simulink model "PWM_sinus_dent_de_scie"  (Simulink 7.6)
settings: Solver=ode15s  StartTime=0.0  StopTime=0.02  RelTol=1e-3
StopFcn:
  | close all, clc
  | load signaux.mat
  | plot(x(1,:),x(2,:),x(1,:),x(3,:),x(1,:),x(4,:))
  | title('Signal PWM, sinus et dent de scie')
  | axis([0 0.02 -2 6])
  | xlabel('temps')
  | grid
libraries: fl_lib x10, nesl_utility x6, elec_lib x1, simulink x1

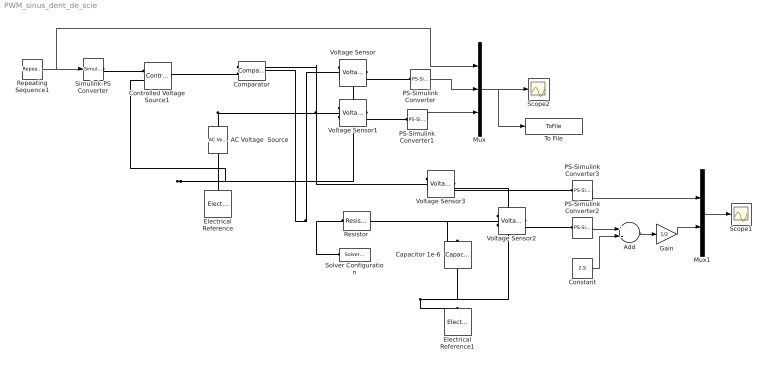
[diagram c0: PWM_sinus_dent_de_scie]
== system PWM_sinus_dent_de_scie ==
  AC Voltage  Source : fl_lib/Electrical/Electrical Sources/AC Voltage Source  DialogController=NetworkEngine.DynNeDlgSource  SystemSampleTime=-1  amp=1 V  shift=0 rad  omega=120 Hz  i_Log=off  v_Log=off  LocalVarNames=|i|v  LocalVarDescs=|i|v  LocalVarLogging=[0 0]
  Add : Sum  Inputs=+-
  Capacitor 1e-6 : fl_lib/Electrical/Electrical Elements/Capacitor  DialogController=NetworkEngine.DynNeDlgSource  SystemSampleTime=-1  c=1e-6 F  v0=0 V  r=1e-6 Ohm  g=0 1/Ohm  i_Log=off  v_Log=off  vc_Log=off  LocalVarNames=|i|v|vc  LocalVarDescs=|i|v|Internal variable for voltage across capacitor term  LocalVarLogging=[0 0 0]
  Comparator : elec_lib/Integrated Circuits/Comparator  DialogController=NetworkEngine.DynNeDlgSource  SystemSampleTime=-1  V_OS=5 mV  V_OL=0 V  V_OH=5 V  C_IN=0 pF  R_OUT=50 Ohm  Delay=0 s  LocalVarLogging=[]
  Constant : Constant  Value=2.5
  Controlled Voltage Source1 : fl_lib/Electrical/Electrical Sources/Controlled Voltage Source  DialogController=NetworkEngine.DynNeDlgSource  SystemSampleTime=-1  i_Log=off  v_Log=off  LocalVarNames=|i|v  LocalVarDescs=|i|v  LocalVarLogging=[0 0]
  Electrical Reference : fl_lib/Electrical/Electrical Elements/Electrical Reference  DialogController=NetworkEngine.DynNeDlgSource  SystemSampleTime=-1  i_Log=off  LocalVarNames=|i  LocalVarDescs=|i  LocalVarLogging=0
  Electrical Reference1 : fl_lib/Electrical/Electrical Elements/Electrical Reference  DialogController=NetworkEngine.DynNeDlgSource  SystemSampleTime=-1  i_Log=off  LocalVarNames=|i  LocalVarDescs=|i  LocalVarLogging=0
  Gain : Gain  Gain=1/2
  Mux : Mux  Inputs=3
  Mux1 : Mux  Inputs=2
  PS-Simulink Converter{,1..3} (4 alike) : nesl_utility/PS-Simulink Converter  DialogController=NetworkEngine.DynNeUtilDlgSource  SystemSampleTime=-1  PhysicalDomain=network_engine_domain  LeftPortType=input  RightPortType=output  SubClassName=ps_output  Unit=1  AffineConversion=off
  Repeating Sequence1 : simulink/Sources/Repeating Sequence  SystemSampleTime=-1  rep_seq_t=[0 0.001]  rep_seq_y=[-1.2 1.2]
  Resistor : fl_lib/Electrical/Electrical Elements/Resistor  DialogController=NetworkEngine.DynNeDlgSource  SystemSampleTime=-1  R=1 kOhm  i_Log=off  v_Log=off  LocalVarNames=|i|v  LocalVarDescs=|i|v  LocalVarLogging=[0 0]
  Scope1 : Scope
  Scope2 : Scope
  Simulink-PS Converter : nesl_utility/Simulink-PS Converter  DialogController=NetworkEngine.DynNeUtilDlgSource  SystemSampleTime=-1  PhysicalDomain=network_engine_domain  LeftPortType=input  RightPortType=output  SubClassName=ps_input  Unit=1  AffineConversion=off  InputFilterTimeConstant=.001  UdotUserProvided=0
  Solver Configuration : nesl_utility/Solver Configuration  DialogController=NetworkEngine.DynNeUtilDlgSource  SystemSampleTime=-1  PhysicalDomain=network_engine_domain  LeftPortType=input  RightPortType=generic  SubClassName=solver  Accelerate=off  Profile=off  ResidualTolerance=1e-9  MaxNonlinIter=12  MaxModeIter=2  DoFixedCost=off  UseLocalSampling=off  DoDC=off  LinearAlgebra=Sparse  LocalSolverSampleTime=.001  LocalSolverChoice=NE_BACKWARD_EULER_ADVANCER  UseLocalSolver=off
  To File : ToFile  Filename=signaux  MatrixName=x
  Voltage Sensor{,1..3} (4 alike) : fl_lib/Electrical/Electrical Sensors/Voltage Sensor  DialogController=NetworkEngine.DynNeDlgSource  SystemSampleTime=-1  i1_Log=off  v1_Log=off  LocalVarNames=|i1|v1  LocalVarDescs=|i1|v1  LocalVarLogging=[0 0]
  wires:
  Repeating Sequence1/1 -> Simulink-PS Converter/1, Mux/1
  Mux/1 -> Scope2/1, To File/1
  PS-Simulink Converter1/1 -> Mux/3
  PS-Simulink Converter/1 -> Mux/2
  PS-Simulink Converter3/1 -> Mux1/1
  Mux1/1 -> Scope1/1
  PS-Simulink Converter2/1 -> Add/1
  Constant/1 -> Add/2
  Gain/1 -> Mux1/2
  Add/1 -> Gain/1
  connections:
  Simulink-PS Converter/RConn1 -- Controlled Voltage Source1/RConn1
  Voltage Sensor/RConn1 -- PS-Simulink Converter/LConn1
  Voltage Sensor1/RConn1 -- PS-Simulink Converter1/LConn1
  Resistor/RConn1 -- Capacitor 1e-6/LConn1 -- Voltage Sensor2/LConn1
  Voltage Sensor2/RConn2 -- Capacitor 1e-6/RConn1 -- Electrical Reference1/LConn1 -- Voltage Sensor3/RConn2
  AC Voltage  Source/LConn1 -- Comparator/LConn1 -- Voltage Sensor1/LConn1 -- Voltage Sensor3/LConn1
  Voltage Sensor2/RConn1 -- PS-Simulink Converter2/LConn1
  Controlled Voltage Source1/LConn1 -- Comparator/LConn2
  Solver Configuration/RConn1 -- Comparator/RConn1 -- Voltage Sensor/LConn1 -- Resistor/LConn1
  Voltage Sensor3/RConn1 -- PS-Simulink Converter3/LConn1
  Voltage Sensor1/RConn2 -- Controlled Voltage Source1/RConn2 -- AC Voltage  Source/RConn1 -- Electrical Reference/LConn1 -- Voltage Sensor/RConn2
